| IBIS file stm32l0_71_72_73_81_82_83_bga100.ibs
| Created by s2ibis version 1.1 (customized version)
| North Carolina State University, ERL, 2006
[IBIS ver] 4.2
[File name] stm32l0_71_72_73_81_82_83_bga100.ibs
[File Rev] 1.0
[Date]  14-03-2016
[Source] Data Created at STMicroelectronics
[Notes]  File originated from ELDO simulations.
[Disclaimer]  This information is for modeling purpose only and is
   not guaranted. The information is subject to change without
   notice.
[Copyright] Copyright 2016 STMicroelectronics Inc.
|   Component stm32l0_71_72_73_81_82_83_bga100
[Component] stm32l0_71_72_73_81_82_83_bga100
[Manufacturer] STMicroelectronics
[Package]
| variable   typ   min   max
R_pkg   0.0   0.0   0.0
L_pkg   0.0H   0.0H   0.0H
C_pkg   0.0F   0.0F   0.0F
[Pin]  signal_name   model_name   R_pin   L_pin   C_pin
B2 PE2 io8p_wsudq_lcd4_ls_ft
A1 PE3 io8p_wsudq_lcd4_ls_ft
B1 PE4 io8p_sudq_ls_ft
C2 PE5 io8p_sudq_ls_ft
D2 PE6 io8p_wsudq_ls_ft_v33
E2 VLCD POWER
C1 PC13 io8p_wsudq_ls_ft_v33
D1 PC14-OSC32_IN io8p_wsudq_ls_ft_v33
E1 PC15-OSC32_OUT io8p_sudq_ls_tc_esdft
F2 PH9 io8p_sudq_ls_ft
G2 PH10 io8p_sudq_ls_ft
F1 PH0-OSC_IN io8p_sudq_ls_tc_esdft
G1 PH1-OSC_OUT io8p_sudq_ls_tc_esdft
H2 NRST ioreset_ft_v33
H1 PC0 io8p_sudq_lcd4_i2cin_ls_ft
J2 PC1 io8p_sudq_lcd4_i2cin_ls_ft
J3 PC2 io8p_wsudq_lcd4_ls_ft
K2 PC3 io8p_wsudq_lcd4_ls_ft
J1 VSSA GND
K1 VREF- GND
L1 VREF+ POWER
M1 VDDA POWER
L2 PA0 io8p_wsudq_ls_ft_v33
M2 PA1 io8p_wsudq_lcd4_ls_ft
K3 PA2 io8p_wsudq_lcd4_ls_ft
L3 PA3 io8p_wsudq_lcd4_ls_ft
E3 VSS GND
H3 VDD POWER
M3 PA4 io8p_wsudq_i2cin_ls_ft
K4 PA5 io8p_wsudq_i2cin_ls_ft
L4 PA6 io8p_wsudq_lcd4_ls_ft
M4 PA7 io8p_wsudq_lcd4_ls_ft
K5 PC4 io8p_wsudq_lcd4_ls_ft
L5 PC5 io8p_wsudq_lcd4_ls_ft
M5 PB0 io8p_wsudq_lcd4_ls_ft
M6 PB1 io8p_wsudq_lcd4_ls_ft
L6 PB2 io8p_wsudq_lcd4_ls_ft
M7 PE7 io8p_wsudq_lcd4_ls_ft
L7 PE8 io8p_wsudq_lcd4_ls_ft
M8 PE9 io8p_wsudq_lcd4_ls_ft
L8 PE10 io8p_wsudq_lcd4_ls_ft
M9 PE11 io8p_wsudq_lcd4_ls_ft
L9 PE12 io8p_wsudq_lcd4_ls_ft
M10 PE13 io8p_wsudq_lcd4_ls_ft
M11 PE14 io8p_wsudq_lcd4_ls_ft
M12 PE15 io8p_wsudq_lcd4_ls_ft
L10 PB10 io8p_sudq_lcd4_i2cin_ls_ft
L11 PB11 io8p_sudq_lcd4_i2cin_ls_ft
F12 VSS GND
G12 VDD POWER
L12 PB12 io8p_wsudq_lcd4_ls_ft
K12 PB13 io8p_sudq_lcd4_i2cin_ls_ft
K11 PB14 io8p_sudq_lcd4_i2cin_ls_ft
K10 PB15 io8p_wsudq_lcd4_ls_ft
K9 PD8 io8p_wsudq_lcd4_ls_ft
K8 PD9 io8p_wsudq_lcd4_ls_ft
J12 PD10 io8p_wsudq_lcd4_ls_ft
J11 PD11 io8p_wsudq_lcd4_ls_ft
J10 PD12 io8p_wsudq_lcd4_ls_ft
H12 PD13 io8p_wsudq_lcd4_ls_ft
H11 PD14 io8p_wsudq_lcd4_ls_ft
H10 PD15 io8p_wsudq_lcd4_ls_ft
E12 PC6 io8p_wsudq_lcd4_ls_ft
E11 PC7 io8p_wsudq_lcd4_ls_ft
E10 PC8 io8p_wsudq_lcd4_ls_ft
D12 PC9 io8p_sudq_lcd4_i2cin_ls_ft
D11 PA8 io8p_sudq_lcd4_i2cin_ls_ft
D10 PA9 io8p_sudq_lcd4_i2cin_ls_ft
C12 PA10 io8p_sudq_lcd4_i2cin_ls_ft
B12 PA11 io8usb_ls_ft
A12 PA12 io8usb_ls_ft
A11 PA13 io8p_sudq_ls_ft
C11 VDD POWER
F11 VSS GND
G11 VDD_USB POWER
A10 PA14 io8p_sudq_ls_ft
A9 PA15 io8p_wsudq_lcd4_ls_ft
B11 PC10 io8p_wsudq_lcd4_ls_ft
C10 PC11 io8p_wsudq_lcd4_ls_ft
B10 PC12 io8p_wsudq_lcd4_ls_ft
C9 PD0 io8p_sudq_ls_ft
B9 PD1 io8p_sudq_ls_ft
C8 PD2 io8p_wsudq_lcd4_ls_ft
B8 PD3 io8p_wsudq_lcd4_ls_ft
B7 PD4 io8p_sudq_ls_ft
A6 PD5 io8p_sudq_ls_ft
B6 PD6 io8p_sudq_ls_ft
A5 PD7 io8p_sudq_ls_ft
A8 PB3 io8p_wsudq_lcd4_ls_ft
A7 PB4 io8p_sudq_lcd4_i2cin_ls_ft
C5 PB5 io8p_wsudq_lcd4_ls_ft
B5 PB6 io8p_wsudq_i2cin_ls_ft
B4 PB7 io8p_wsudq_i2cin_ls_ft
A4 BOOT0 vpp_test_hv
A3 PB8 io8p_sudq_lcd4_i2cin_ls_ft
B3 PB9 io8p_sudq_lcd4_i2cin_ls_ft
C3 PE0 io8p_wsudq_lcd4_ls_ft
A2 PE1 io8p_wsudq_lcd4_ls_ft
D3 VSS GND
C4 VDD POWER
[Model Selector] io8p_sudq_ls_ft
io8p00_sudq_ls_ft_pd_lv  "SPEED00 1P8V, PD=40kOhm"
io8p00_sudq_ls_ft_pu_lv  "SPEED00 1P8V, PU=40kOhm"
io8p00_sudq_ls_ft_lv  "SPEED00 1P8V"
io8p01_sudq_ls_ft_pd_lv  "SPEED01 1P8V, PD=40kOhm"
io8p01_sudq_ls_ft_pu_lv  "SPEED01 1P8V, PU=40kOhm"
io8p01_sudq_ls_ft_lv  "SPEED01 1P8V"
io8p10_sudq_ls_ft_pd_lv  "SPEED10 1P8V, PD=40kOhm"
io8p10_sudq_ls_ft_pu_lv  "SPEED10 1P8V, PU=40kOhm"
io8p10_sudq_ls_ft_lv  "SPEED10 1P8V"
io8p11_sudq_ls_ft_pd_lv  "SPEED11 1P8V, PD=40kOhm"
io8p11_sudq_ls_ft_pu_lv  "SPEED11 1P8V, PU=40kOhm"
io8p11_sudq_ls_ft_lv  "SPEED11 1P8V"
io8p00_sudq_ls_ft_pd  "SPEED00, PD=40kOhm"
io8p00_sudq_ls_ft_pu  "SPEED00, PU=40kOhm"
io8p00_sudq_ls_ft  "SPEED00"
io8p01_sudq_ls_ft_pd  "SPEED01, PD=40kOhm"
io8p01_sudq_ls_ft_pu  "SPEED01, PU=40kOhm"
io8p01_sudq_ls_ft  "SPEED01"
io8p10_sudq_ls_ft_pd  "SPEED10, PD=40kOhm"
io8p10_sudq_ls_ft_pu  "SPEED10, PU=40kOhm"
io8p10_sudq_ls_ft  "SPEED10"
io8p11_sudq_ls_ft_pd  "SPEED11, PD=40kOhm"
io8p11_sudq_ls_ft_pu  "SPEED11, PU=40kOhm"
io8p11_sudq_ls_ft  "SPEED11"
[Model Selector] io8p_sudq_ls_tc_esdft
io8p00_sudq_ls_tc_esdft_pd_lv  "SPEED00 1P8V, PD=40kOhm"
io8p00_sudq_ls_tc_esdft_pu_lv  "SPEED00 1P8V, PU=40kOhm"
io8p00_sudq_ls_tc_esdft_lv  "SPEED00 1P8V"
io8p01_sudq_ls_tc_esdft_pd_lv  "SPEED01 1P8V, PD=40kOhm"
io8p01_sudq_ls_tc_esdft_pu_lv  "SPEED01 1P8V, PU=40kOhm"
io8p01_sudq_ls_tc_esdft_lv  "SPEED01 1P8V"
io8p10_sudq_ls_tc_esdft_pd_lv  "SPEED10 1P8V, PD=40kOhm"
io8p10_sudq_ls_tc_esdft_pu_lv  "SPEED10 1P8V, PU=40kOhm"
io8p10_sudq_ls_tc_esdft_lv  "SPEED10 1P8V"
io8p11_sudq_ls_tc_esdft_pd_lv  "SPEED11 1P8V, PD=40kOhm"
io8p11_sudq_ls_tc_esdft_pu_lv  "SPEED11 1P8V, PU=40kOhm"
io8p11_sudq_ls_tc_esdft_lv  "SPEED11 1P8V"
io8p00_sudq_ls_tc_esdft_pd  "SPEED00, PD=40kOhm"
io8p00_sudq_ls_tc_esdft_pu  "SPEED00, PU=40kOhm"
io8p00_sudq_ls_tc_esdft  "SPEED00"
io8p01_sudq_ls_tc_esdft_pd  "SPEED01, PD=40kOhm"
io8p01_sudq_ls_tc_esdft_pu  "SPEED01, PU=40kOhm"
io8p01_sudq_ls_tc_esdft  "SPEED01"
io8p10_sudq_ls_tc_esdft_pd  "SPEED10, PD=40kOhm"
io8p10_sudq_ls_tc_esdft_pu  "SPEED10, PU=40kOhm"
io8p10_sudq_ls_tc_esdft  "SPEED10"
io8p11_sudq_ls_tc_esdft_pd  "SPEED11, PD=40kOhm"
io8p11_sudq_ls_tc_esdft_pu  "SPEED11, PU=40kOhm"
io8p11_sudq_ls_tc_esdft  "SPEED11"
[Model Selector] io8p_wsudq_i2cin_ls_ft
io8p00_wsudq_i2cin_ls_ft_pd_lv  "SPEED00 1P8V, PD=40kOhm"
io8p00_wsudq_i2cin_ls_ft_pu_lv  "SPEED00 1P8V, PU=40kOhm"
io8p00_wsudq_i2cin_ls_ft_lv  "SPEED00 1P8V"
io8p01_wsudq_i2cin_ls_ft_pd_lv  "SPEED01 1P8V, PD=40kOhm"
io8p01_wsudq_i2cin_ls_ft_pu_lv  "SPEED01 1P8V, PU=40kOhm"
io8p01_wsudq_i2cin_ls_ft_lv  "SPEED01 1P8V"
io8p10_wsudq_i2cin_ls_ft_pd_lv  "SPEED10 1P8V, PD=40kOhm"
io8p10_wsudq_i2cin_ls_ft_pu_lv  "SPEED10 1P8V, PU=40kOhm"
io8p10_wsudq_i2cin_ls_ft_lv  "SPEED10 1P8V"
io8p11_wsudq_i2cin_ls_ft_pd_lv  "SPEED11 1P8V, PD=40kOhm"
io8p11_wsudq_i2cin_ls_ft_pu_lv  "SPEED11 1P8V, PU=40kOhm"
io8p11_wsudq_i2cin_ls_ft_lv  "SPEED11 1P8V"
io8p00_wsudq_i2cin_ls_ft_pd  "SPEED00, PD=40kOhm"
io8p00_wsudq_i2cin_ls_ft_pu  "SPEED00, PU=40kOhm"
io8p00_wsudq_i2cin_ls_ft  "SPEED00"
io8p01_wsudq_i2cin_ls_ft_pd  "SPEED01, PD=40kOhm"
io8p01_wsudq_i2cin_ls_ft_pu  "SPEED01, PU=40kOhm"
io8p01_wsudq_i2cin_ls_ft  "SPEED01"
io8p10_wsudq_i2cin_ls_ft_pd  "SPEED10, PD=40kOhm"
io8p10_wsudq_i2cin_ls_ft_pu  "SPEED10, PU=40kOhm"
io8p10_wsudq_i2cin_ls_ft  "SPEED10"
io8p11_wsudq_i2cin_ls_ft_pd  "SPEED11, PD=40kOhm"
io8p11_wsudq_i2cin_ls_ft_pu  "SPEED11, PU=40kOhm"
io8p11_wsudq_i2cin_ls_ft  "SPEED11"
[Model Selector] io8p_wsudq_lcd4_ls_ft
io8p00_wsudq_lcd4_ls_ft_pd_lv  "SPEED00 1P8V, PD=40kOhm"
io8p00_wsudq_lcd4_ls_ft_pu_lv  "SPEED00 1P8V, PU=40kOhm"
io8p00_wsudq_lcd4_ls_ft_lv  "SPEED00 1P8V"
io8p01_wsudq_lcd4_ls_ft_pd_lv  "SPEED01 1P8V, PD=40kOhm"
io8p01_wsudq_lcd4_ls_ft_pu_lv  "SPEED01 1P8V, PU=40kOhm"
io8p01_wsudq_lcd4_ls_ft_lv  "SPEED01 1P8V"
io8p10_wsudq_lcd4_ls_ft_pd_lv  "SPEED10 1P8V, PD=40kOhm"
io8p10_wsudq_lcd4_ls_ft_pu_lv  "SPEED10 1P8V, PU=40kOhm"
io8p10_wsudq_lcd4_ls_ft_lv  "SPEED10 1P8V"
io8p11_wsudq_lcd4_ls_ft_pd_lv  "SPEED11 1P8V, PD=40kOhm"
io8p11_wsudq_lcd4_ls_ft_pu_lv  "SPEED11 1P8V, PU=40kOhm"
io8p11_wsudq_lcd4_ls_ft_lv  "SPEED11 1P8V"
io8p00_wsudq_lcd4_ls_ft_pd  "SPEED00, PD=40kOhm"
io8p00_wsudq_lcd4_ls_ft_pu  "SPEED00, PU=40kOhm"
io8p00_wsudq_lcd4_ls_ft  "SPEED00"
io8p01_wsudq_lcd4_ls_ft_pd  "SPEED01, PD=40kOhm"
io8p01_wsudq_lcd4_ls_ft_pu  "SPEED01, PU=40kOhm"
io8p01_wsudq_lcd4_ls_ft  "SPEED01"
io8p10_wsudq_lcd4_ls_ft_pd  "SPEED10, PD=40kOhm"
io8p10_wsudq_lcd4_ls_ft_pu  "SPEED10, PU=40kOhm"
io8p10_wsudq_lcd4_ls_ft  "SPEED10"
io8p11_wsudq_lcd4_ls_ft_pd  "SPEED11, PD=40kOhm"
io8p11_wsudq_lcd4_ls_ft_pu  "SPEED11, PU=40kOhm"
io8p11_wsudq_lcd4_ls_ft  "SPEED11"
[Model Selector] io8p_wsudq_ls_ft_v33
io8p00_wsudq_ls_ft_v33_pd_lv  "SPEED00 1P8V, PD=40kOhm"
io8p00_wsudq_ls_ft_v33_pu_lv  "SPEED00 1P8V, PU=40kOhm"
io8p00_wsudq_ls_ft_v33_lv  "SPEED00 1P8V"
io8p01_wsudq_ls_ft_v33_pd_lv  "SPEED01 1P8V, PD=40kOhm"
io8p01_wsudq_ls_ft_v33_pu_lv  "SPEED01 1P8V, PU=40kOhm"
io8p01_wsudq_ls_ft_v33_lv  "SPEED01 1P8V"
io8p10_wsudq_ls_ft_v33_pd_lv  "SPEED10 1P8V, PD=40kOhm"
io8p10_wsudq_ls_ft_v33_pu_lv  "SPEED10 1P8V, PU=40kOhm"
io8p10_wsudq_ls_ft_v33_lv  "SPEED10 1P8V"
io8p11_wsudq_ls_ft_v33_pd_lv  "SPEED11 1P8V, PD=40kOhm"
io8p11_wsudq_ls_ft_v33_pu_lv  "SPEED11 1P8V, PU=40kOhm"
io8p11_wsudq_ls_ft_v33_lv  "SPEED11 1P8V"
io8p00_wsudq_ls_ft_v33_pd  "SPEED00, PD=40kOhm"
io8p00_wsudq_ls_ft_v33_pu  "SPEED00, PU=40kOhm"
io8p00_wsudq_ls_ft_v33  "SPEED00"
io8p01_wsudq_ls_ft_v33_pd  "SPEED01, PD=40kOhm"
io8p01_wsudq_ls_ft_v33_pu  "SPEED01, PU=40kOhm"
io8p01_wsudq_ls_ft_v33  "SPEED01"
io8p10_wsudq_ls_ft_v33_pd  "SPEED10, PD=40kOhm"
io8p10_wsudq_ls_ft_v33_pu  "SPEED10, PU=40kOhm"
io8p10_wsudq_ls_ft_v33  "SPEED10"
io8p11_wsudq_ls_ft_v33_pd  "SPEED11, PD=40kOhm"
io8p11_wsudq_ls_ft_v33_pu  "SPEED11, PU=40kOhm"
io8p11_wsudq_ls_ft_v33  "SPEED11"
[Model Selector] vpp_test_hv
vpp_test_hv_2p4  "Input Buffer 1P65V"
vpp_test_hv_3p3  "Input Buffer"
[Model Selector] io8usb_ls_ft
io8usb_ls_ft_dpdn_pu  "HS USB DP/DN IO + PU=1.2kOhm"
io8usb_ls_ft_dpdn  "HS USB DP/DN IO"
io8p00_ls_ft_pd_lv  "SPEED00 1P8V, PD=40kOhm"
io8p00_ls_ft_pu_lv  "SPEED00 1P8V, PU=40kOhm"
io8p00_ls_ft_lv  "SPEED00 1P8V"
io8p01_ls_ft_pd_lv  "SPEED01 1P8V, PD=40kOhm"
io8p01_ls_ft_pu_lv  "SPEED01 1P8V, PU=40kOhm"
io8p01_ls_ft_lv  "SPEED01 1P8V"
io8p10_ls_ft_pd_lv  "SPEED10 1P8V, PD=40kOhm"
io8p10_ls_ft_pu_lv  "SPEED10 1P8V, PU=40kOhm"
io8p10_ls_ft_lv  "SPEED10 1P8V"
io8p11_ls_ft_pd_lv  "SPEED11 1P8V, PD=40kOhm"
io8p11_ls_ft_pu_lv  "SPEED11 1P8V, PU=40kOhm"
io8p11_ls_ft_lv  "SPEED11 1P8V"
io8p00_ls_ft_pd  "SPEED00, PD=40kOhm"
io8p00_ls_ft_pu  "SPEED00, PU=40kOhm"
io8p00_ls_ft  "SPEED00"
io8p01_ls_ft_pd  "SPEED01, PD=40kOhm"
io8p01_ls_ft_pu  "SPEED01, PU=40kOhm"
io8p01_ls_ft  "SPEED01"
io8p10_ls_ft_pd  "SPEED10, PD=40kOhm"
io8p10_ls_ft_pu  "SPEED10, PU=40kOhm"
io8p10_ls_ft  "SPEED10"
io8p11_ls_ft_pd  "SPEED11, PD=40kOhm"
io8p11_ls_ft_pu  "SPEED11, PU=40kOhm"
io8p11_ls_ft  "SPEED11"
[Model Selector] io8p_sudq_lcd4_i2cin_ls_ft
io8p00_sudq_lcd4_i2cin_ls_ft_pd_lv  "SPEED00 1P8V, PD=40kOhm"
io8p00_sudq_lcd4_i2cin_ls_ft_pu_lv  "SPEED00 1P8V, PU=40kOhm"
io8p00_sudq_lcd4_i2cin_ls_ft_lv  "SPEED00 1P8V"
io8p01_sudq_lcd4_i2cin_ls_ft_pd_lv  "SPEED01 1P8V, PD=40kOhm"
io8p01_sudq_lcd4_i2cin_ls_ft_pu_lv  "SPEED01 1P8V, PU=40kOhm"
io8p01_sudq_lcd4_i2cin_ls_ft_lv  "SPEED01 1P8V"
io8p10_sudq_lcd4_i2cin_ls_ft_pd_lv  "SPEED10 1P8V, PD=40kOhm"
io8p10_sudq_lcd4_i2cin_ls_ft_pu_lv  "SPEED10 1P8V, PU=40kOhm"
io8p10_sudq_lcd4_i2cin_ls_ft_lv  "SPEED10 1P8V"
io8p11_sudq_lcd4_i2cin_ls_ft_pd_lv  "SPEED11 1P8V, PD=40kOhm"
io8p11_sudq_lcd4_i2cin_ls_ft_pu_lv  "SPEED11 1P8V, PU=40kOhm"
io8p11_sudq_lcd4_i2cin_ls_ft_lv  "SPEED11 1P8V"
io8p00_sudq_lcd4_i2cin_ls_ft_pd  "SPEED00, PD=40kOhm"
io8p00_sudq_lcd4_i2cin_ls_ft_pu  "SPEED00, PU=40kOhm"
io8p00_sudq_lcd4_i2cin_ls_ft  "SPEED00"
io8p01_sudq_lcd4_i2cin_ls_ft_pd  "SPEED01, PD=40kOhm"
io8p01_sudq_lcd4_i2cin_ls_ft_pu  "SPEED01, PU=40kOhm"
io8p01_sudq_lcd4_i2cin_ls_ft  "SPEED01"
io8p10_sudq_lcd4_i2cin_ls_ft_pd  "SPEED10, PD=40kOhm"
io8p10_sudq_lcd4_i2cin_ls_ft_pu  "SPEED10, PU=40kOhm"
io8p10_sudq_lcd4_i2cin_ls_ft  "SPEED10"
io8p11_sudq_lcd4_i2cin_ls_ft_pd  "SPEED11, PD=40kOhm"
io8p11_sudq_lcd4_i2cin_ls_ft_pu  "SPEED11, PU=40kOhm"
io8p11_sudq_lcd4_i2cin_ls_ft  "SPEED11"
[Model Selector] ioreset_ft_v33
ioreset_ft_v33_pu_lv  "ioreset 1P8V + PU=40kOhm"
ioreset_ft_v33_nopu_lv  "ioreset 1P8V"
ioreset_ft_v33_pu  "ioreset + PU=40kOhm"
ioreset_ft_v33_nopu  "ioreset"
| Models and submodels in the file (176): io8p00_sudq_ls_ft_pd_lv (I/O), io8p00_sudq_ls_ft_pu_lv (I/O), io8p00_sudq_ls_ft_lv (I/O), io8p01_sudq_ls_ft_pd_lv (I/O), io8p01_sudq_ls_ft_pu_lv (I/O), io8p01_sudq_ls_ft_lv (I/O), io8p10_sudq_ls_ft_pd_lv (I/O), io8p10_sudq_ls_ft_pu_lv (I/O), io8p10_sudq_ls_ft_lv (I/O), io8p11_sudq_ls_ft_pd_lv (I/O), io8p11_sudq_ls_ft_pu_lv (I/O), io8p11_sudq_ls_ft_lv (I/O), io8p00_sudq_ls_ft_pd (I/O), io8p00_sudq_ls_ft_pu (I/O), io8p00_sudq_ls_ft (I/O), io8p01_sudq_ls_ft_pd (I/O), io8p01_sudq_ls_ft_pu (I/O), io8p01_sudq_ls_ft (I/O), io8p10_sudq_ls_ft_pd (I/O), io8p10_sudq_ls_ft_pu (I/O), io8p10_sudq_ls_ft (I/O), io8p11_sudq_ls_ft_pd (I/O), io8p11_sudq_ls_ft_pu (I/O), io8p11_sudq_ls_ft (I/O), io8p00_sudq_ls_tc_esdft_pd_lv (I/O), io8p00_sudq_ls_tc_esdft_pu_lv (I/O), io8p00_sudq_ls_tc_esdft_lv (I/O), io8p01_sudq_ls_tc_esdft_pd_lv (I/O), io8p01_sudq_ls_tc_esdft_pu_lv (I/O), io8p01_sudq_ls_tc_esdft_lv (I/O), io8p10_sudq_ls_tc_esdft_pd_lv (I/O), io8p10_sudq_ls_tc_esdft_pu_lv (I/O), io8p10_sudq_ls_tc_esdft_lv (I/O), io8p11_sudq_ls_tc_esdft_pd_lv (I/O), io8p11_sudq_ls_tc_esdft_pu_lv (I/O), io8p11_sudq_ls_tc_esdft_lv (I/O), io8p00_sudq_ls_tc_esdft_pd (I/O), io8p00_sudq_ls_tc_esdft_pu (I/O), io8p00_sudq_ls_tc_esdft (I/O), io8p01_sudq_ls_tc_esdft_pd (I/O), io8p01_sudq_ls_tc_esdft_pu (I/O), io8p01_sudq_ls_tc_esdft (I/O), io8p10_sudq_ls_tc_esdft_pd (I/O), io8p10_sudq_ls_tc_esdft_pu (I/O), io8p10_sudq_ls_tc_esdft (I/O), io8p11_sudq_ls_tc_esdft_pd (I/O), io8p11_sudq_ls_tc_esdft_pu (I/O), io8p11_sudq_ls_tc_esdft (I/O), io8p00_wsudq_i2cin_ls_ft_pd_lv (I/O), io8p00_wsudq_i2cin_ls_ft_pu_lv (I/O), io8p00_wsudq_i2cin_ls_ft_lv (I/O), io8p01_wsudq_i2cin_ls_ft_pd_lv (I/O), io8p01_wsudq_i2cin_ls_ft_pu_lv (I/O), io8p01_wsudq_i2cin_ls_ft_lv (I/O), io8p10_wsudq_i2cin_ls_ft_pd_lv (I/O), io8p10_wsudq_i2cin_ls_ft_pu_lv (I/O), io8p10_wsudq_i2cin_ls_ft_lv (I/O), io8p11_wsudq_i2cin_ls_ft_pd_lv (I/O), io8p11_wsudq_i2cin_ls_ft_pu_lv (I/O), io8p11_wsudq_i2cin_ls_ft_lv (I/O), io8p00_wsudq_i2cin_ls_ft_pd (I/O), io8p00_wsudq_i2cin_ls_ft_pu (I/O), io8p00_wsudq_i2cin_ls_ft (I/O), io8p01_wsudq_i2cin_ls_ft_pd (I/O), io8p01_wsudq_i2cin_ls_ft_pu (I/O), io8p01_wsudq_i2cin_ls_ft (I/O), io8p10_wsudq_i2cin_ls_ft_pd (I/O), io8p10_wsudq_i2cin_ls_ft_pu (I/O), io8p10_wsudq_i2cin_ls_ft (I/O), io8p11_wsudq_i2cin_ls_ft_pd (I/O), io8p11_wsudq_i2cin_ls_ft_pu (I/O), io8p11_wsudq_i2cin_ls_ft (I/O), io8p00_wsudq_lcd4_ls_ft_pd_lv (I/O), io8p00_wsudq_lcd4_ls_ft_pu_lv (I/O), io8p00_wsudq_lcd4_ls_ft_lv (I/O), io8p01_wsudq_lcd4_ls_ft_pd_lv (I/O), io8p01_wsudq_lcd4_ls_ft_pu_lv (I/O), io8p01_wsudq_lcd4_ls_ft_lv (I/O), io8p10_wsudq_lcd4_ls_ft_pd_lv (I/O), io8p10_wsudq_lcd4_ls_ft_pu_lv (I/O)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
